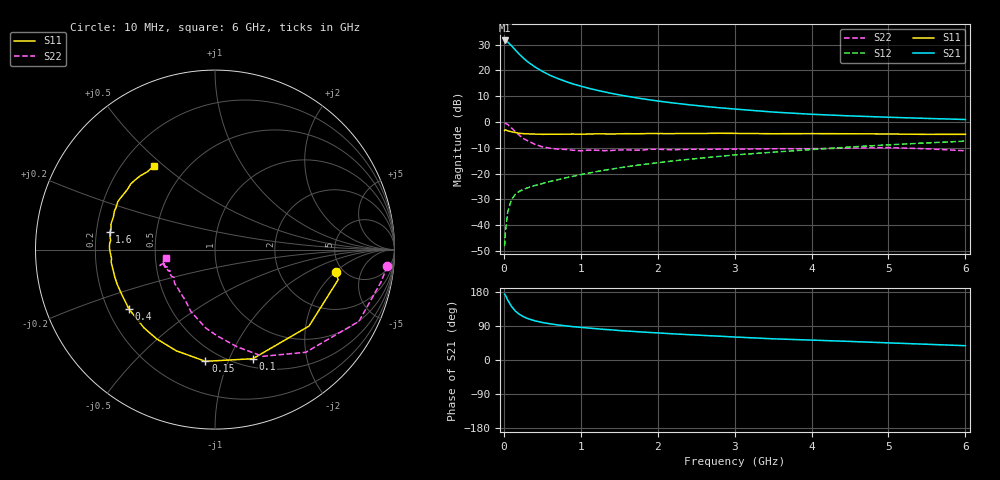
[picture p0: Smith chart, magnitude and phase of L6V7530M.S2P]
!  INFINEON TECHNOLOGIES Small Signal Semiconductors
! BFR380L3 , Si-NPN RF-Transistor in TSLP-3-1
!  Vce=0.75 V,  Ic=30 mA
! Common Emitter S-Parameters:  07. March 2005
#  GHz  S  MA  R  50
! f  S11  S21  S12  S22
! GHz  Mag  Ang  Mag  Ang  Mag  Ang  Mag  Ang
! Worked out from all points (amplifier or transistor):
!   36 points, 10 MHz to 6 GHz, reference 50 ohm
!   highest |S21| = 31.6 dB at 10 MHz (marker M1)
!   |S21| within 3 dB of that: start of sweep to 128.5 MHz
!   unconditionally stable (mu >= 1): 1.526 GHz to 5.701 GHz
!   at 250 MHz: K = 0.44, MSG = 25.6 dB, |S12| = -26.2 dB
!   at 1.4 GHz: K = 0.99, MSG = 14.7 dB, |S12| = -18.3 dB
!   at 6 GHz: K = 1.00, MSG = 4.2 dB, |S12| = -7.4 dB
!   S11 on the Smith chart (normalised r, x): 10 MHz: 4.30, -2.05; 100 MHz: 0.59, -1.22; 150 MHz: 0.41, -0.83; 400 MHz: 0.29, -0.29; 1.6 GHz: 0.26, +0.08; 6 GHz: 0.33, +0.47
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0.01  0.6838 -10.7  38.14 173.7  0.0039 75.4  0.9647 -5.4
0.02  0.7065 -13.7  37.72 171.3  0.0074 83.2  0.9422 -11.1
0.05  0.6753 -39.1  35.58 158.4  0.0179 74.1  0.896 -26.5
0.1  0.6434 -70.9  30.08 141.4  0.0315 61.5  0.7637 -48.5
0.15  0.6249 -94.9  24.88 129.1  0.0395 53.5  0.6514 -65.9
0.2  0.6036 -111.0  20.7 120.8  0.0451 50.9  0.5548 -77.3
0.25  0.5942 -123.2  17.59 114.8  0.049 47.9  0.48 -88.7
0.3  0.5888 -132.2  15.1 110.1  0.0522 47.8  0.4395 -96.8
0.4  0.5826 -145.5  11.79 103.5  0.0585 47.8  0.3702 -111.3
0.5  0.5764 -154.1  9.617 99.0  0.0638 50.0  0.3294 -119.8
0.6  0.5782 -160.4  8.046 95.5  0.0703 51.5  0.3106 -127.3
0.7  0.5789 -164.8  6.976 92.7  0.0758 53.5  0.2982 -134.2
0.9  0.5829 -173.1  5.459 88.0  0.0883 56.6  0.2836 -144.2
1.1  0.5838 -178.2  4.521 84.3  0.1019 58.7  0.2846 -148.7
1.3  0.5878 176.5  3.861 80.8  0.1158 60.0  0.2777 -155.2
1.6  0.5942 170.7  3.156 76.4  0.1358 61.0  0.2878 -159.7
2.2  0.5948 161.8  2.341 69.0  0.1754 62.1  0.2892 -161.6
2.8  0.6039 153.7  1.89 62.8  0.2149 62.2  0.2978 -165.6
3.5  0.5919 145.5  1.558 55.9  0.2596 60.2  0.3026 -164.9
4.5  0.591 139.2  1.312 49.0  0.3266 58.1  0.3112 -164.5
5.5  0.5746 131.0  1.172 41.5  0.3927 53.7  0.3019 -165.8
6  0.5768 125.9  1.118 37.7  0.4252 51.4  0.2765 -170.4
